FUNCTION_BLOCK FB44
TITLE =Set All Digital Inputs
//*****************************************************************************
//* maxon motor ag
//* R&D
//* all rights reserved
//*****************************************************************************
//* Summary:  Write all digital inputs
//*
//* Remarks:
//*
//* Created under: STEP7 REV5.2+SP1
//*****************************************************************************
//* History:
//* 18.05.2004 | INA   first release
//*
//*
//*****************************************************************************
//

AUTHOR:INA
FAMILY:I_O_Mode
NAME:SetDigOu
VERSION:00.01


VAR_INPUT

Write : BOOL //A rising edge start the command

  NodeID : BYTE //Adress of the maxon device

  Outputs : WORD //Sets all digital outputs

END_VAR
VAR_OUTPUT
  Done : BOOL //Data valid flag is TRUE if data were available

  Err : BOOL //Error flag is TRUE if an Error has occured, see ErrNo for more details

  ErrNo : DINT //Contains detailed error information

END_VAR
VAR
  xEdgeMerker : BOOL //Edge Merker

  xEdgeFlag : BOOL //Edge Flag

  xStep : INT
END_VAR

BEGIN

NETWORK
TITLE = Activate the service function
//

// SDO Write "Set All digital Inputs

       U    #Write
       FP   #xEdgeFlag                   // recognize a positiv edge of the Read signal
       =    #xEdgeMerker                 // and set the xEdgeMerker for one cycle to true

       L    #xStep
       L    0
       ==I
       U    #xEdgeMerker
       SPB  nstp                         // iStep = 1 -> fnc1

       L    #xStep                       // jump list
       SPL  List
       SPA  rdef
       SPA  fnc1
       SPA  fncE
List  :SPA  rdef

rdef  :NOP  0
       R    #Done                        // reset Done
       R    #Err
       L    0
       T    #xStep                       // iStep = 0
       SPA  end

fnc1  :NOP  0
       CALL FC15
         NodeID:=#NodeID
         Index:=DW#16#00002078
         SubIndex:=DW#16#00000001
         ValueIn:=#Outputs
         RET_VAL:=#Done
         Err:=#Err
         ErrNo:=#ErrNo

fncE  :NOP  0
       L    0
       T    #xStep
       SPA  end

nstp  :NOP  0
       L    #xStep
       INC            1
       T    #xStep

end   :NOP  0
END_FUNCTION_BLOCK
